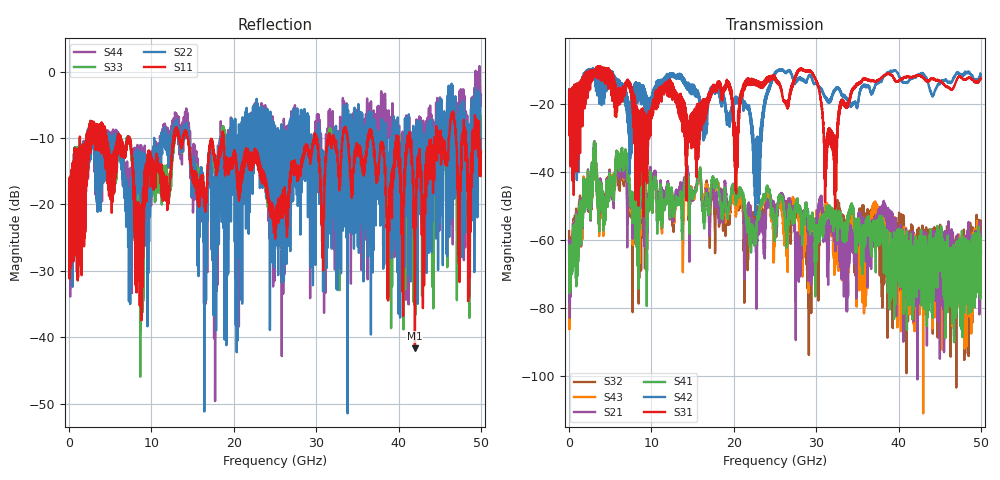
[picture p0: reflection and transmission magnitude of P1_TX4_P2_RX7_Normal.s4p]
!Keysight Technologies,N5225B,MY57041031,A.13.20.10
!Date: Friday, May 31, 2019 11:38:43
!Correction: S11(Full 4 Port(1,2,3,4))
!S12(Full 4 Port(1,2,3,4))
!S13(Full 4 Port(1,2,3,4))
!S14(Full 4 Port(1,2,3,4))
!S21(Full 4 Port(1,2,3,4))
!S22(Full 4 Port(1,2,3,4))
!S23(Full 4 Port(1,2,3,4))
!S24(Full 4 Port(1,2,3,4))
!S31(Full 4 Port(1,2,3,4))
!S32(Full 4 Port(1,2,3,4))
!S33(Full 4 Port(1,2,3,4))
!S34(Full 4 Port(1,2,3,4))
!S41(Full 4 Port(1,2,3,4))
!S42(Full 4 Port(1,2,3,4))
!S43(Full 4 Port(1,2,3,4))
!S44(Full 4 Port(1,2,3,4))
!S4P File: Measurements: <S11,S12,S13,S14>,
!<S21,S22,S23,S24>,
!<S31,S32,S33,S34>,
!<S41,S42,S43,S44>:
# Hz S  dB  R 50.0
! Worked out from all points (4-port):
!   5000 points, 10 MHz to 50 GHz, reference 50 ohm
!   strongest paths, dB at 10 MHz, 12.51 GHz, 25.01 GHz, 37.51 GHz, 50 GHz:
!     S31: -19.5, -17.6, -12.9, -13.1, -12.6
!     S42: -19.5, -12.1, -11.4, -13.8, -11.8
!     S41: -61.7, -45.8, -58.5, -55.6, -59.4
!     S21: -60.2, -48.7, -52.0, -52.7, -64.6
!     S43: -62.7, -47.0, -55.9, -52.4, -60.8
!     S32: -57.4, -50.3, -52.0, -59.0, -63.8
!   lowest |S11| = -41.7 dB at 41.99 GHz (marker M1), VSWR 1.02, Z = 50.8 - j0.279 ohm
!   |S11| at or under -10 dB: 7.336 GHz to 12.7 GHz (5.362 GHz wide, 53.5 % of centre); 14.41 GHz to 18.57 GHz (4.156 GHz wide, 25.2 % of centre); 18.74 GHz to 29.76 GHz (11.02 GHz wide, 45.4 % of centre)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
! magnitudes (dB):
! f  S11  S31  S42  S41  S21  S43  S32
! 10 MHz  -19.5  -19.5  -19.5  -61.7  -60.2  -62.7  -57.4
! 6.64 GHz  -12.3  -15.4  -18.8  -37.0  -38.9  -39.0  -40.7
! 22.8 GHz  -13.0  -13.4  -37.1  -55.7  -68.5  -56.5  -53.5
! 29.18 GHz  -13.0  -10.2  -11.6  -54.5  -63.4  -64.2  -63.5
! 32.24 GHz  -10.4  -35.5  -15.9  -51.0  -57.7  -68.3  -59.9
! 41.99 GHz  -41.7  -11.9  -12.3  -60.0  -64.7  -58.5  -64.8
! 50 GHz  -12.1  -12.6  -11.8  -59.4  -64.6  -60.8  -63.8
